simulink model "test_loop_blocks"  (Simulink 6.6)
settings: Solver=ode45  StartTime=0.0  StopTime=10.0  RelTol=1e-3
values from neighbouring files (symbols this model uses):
  param = params{get(handles.paramList, 'Value')}    [loopgui.m]
undefined symbols (not defined in the file or in its folder): Generator, signal, test_loop_blocks
libraries: sltpda x15

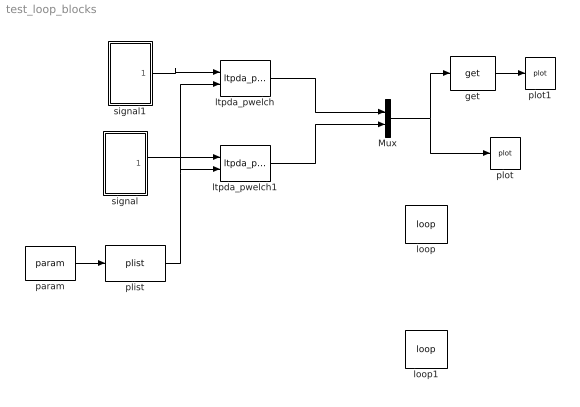
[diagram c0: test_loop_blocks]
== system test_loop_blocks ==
  Mux : Mux  Inputs=2
  get : sltpda/AO class/get  Tag=get  Description=Get the propery of an analysis object.  SystemSampleTime=-1  param=hist
  loop : sltpda/Parameters/loop  SystemSampleTime=-1  block=test_loop_blocks/param  blockHandle=158.001708984375  key=val  vals=500 1000  loopon=on  level=1
  loop1 : sltpda/Parameters/loop  SystemSampleTime=-1  block=test_loop_blocks/signal/Signal Generator  blockHandle=165.0015869140625  key=tsfcn  vals=sin(2*pi*10*t) sin(2*pi*1*t)  loopon=on  level=2
  ltpda_pwelch : sltpda/Signal Processing blocks/Frequency domain/ltpda_pwelch  Tag=ltpda_pwelch  Description=Makes a spectral density estimate by calling ltpda_pwlech.  SystemSampleTime=-1
  ltpda_pwelch1 : sltpda/Signal Processing blocks/Frequency domain/ltpda_pwelch  Tag=ltpda_pwelch  Description=Makes a spectral density estimate by calling ltpda_pwlech.  SystemSampleTime=-1
  param : sltpda/Parameters/param  Tag=param  SystemSampleTime=-1  key=Nfft  val=500
  plist : sltpda/Parameters/plist  SystemSampleTime=-1
  plot : sltpda/Sinks/plot  Tag=plot  Description=Plot an analysis object.  SystemSampleTime=-1  xscale=linear  yscale=linear
  plot1 : sltpda/Sinks/plot  Tag=plot  Description=Plot an analysis object.  SystemSampleTime=-1  xscale=linear  yscale=linear
  signal : Subsystem
  signal1 : Subsystem
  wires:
  Mux/1 -> plot/1, get/1
  signal1/1(Out1) -> ltpda_pwelch/1
  ltpda_pwelch/1 -> Mux/1
  ltpda_pwelch1/1 -> Mux/2
  signal/1(Out1) -> ltpda_pwelch1/1
  param/1 -> plist/1
  plist/1 -> ltpda_pwelch1/2, ltpda_pwelch/2
  get/1 -> plot1/1

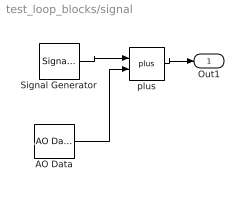
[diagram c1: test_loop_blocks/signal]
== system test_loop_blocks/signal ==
  AO Data : sltpda/Sources/AO Data  Tag=ao  SystemSampleTime=-1  vals=5
  Signal Generator : sltpda/Sources/Signal Generator  Tag=ao  SystemSampleTime=-1  nsecs=20  fs=100  tsfcn=sin(2*pi*10*t)
  plus : sltpda/math blocks/plus  Tag=plus  SystemSampleTime=-1
  Out1 : Outport
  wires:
  Signal Generator/1 -> plus/1
  plus/1 -> Out1/1
  AO Data/1 -> plus/2

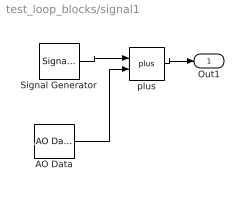
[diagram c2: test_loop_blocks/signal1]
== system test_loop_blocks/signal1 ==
  AO Data : sltpda/Sources/AO Data  Tag=ao  SystemSampleTime=-1  vals=10
  Signal Generator : sltpda/Sources/Signal Generator  Tag=ao  SystemSampleTime=-1  nsecs=20  fs=100  tsfcn=sin(2*pi*10*t)
  plus : sltpda/math blocks/plus  Tag=plus  SystemSampleTime=-1
  Out1 : Outport
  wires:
  AO Data/1 -> plus/2
  plus/1 -> Out1/1
  Signal Generator/1 -> plus/1
